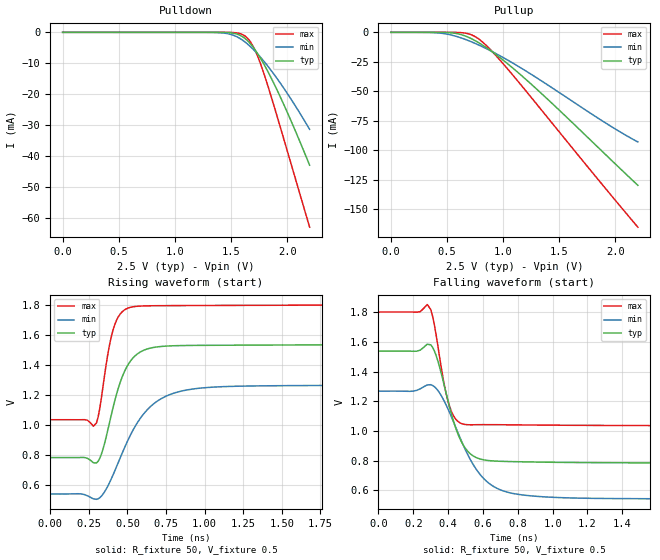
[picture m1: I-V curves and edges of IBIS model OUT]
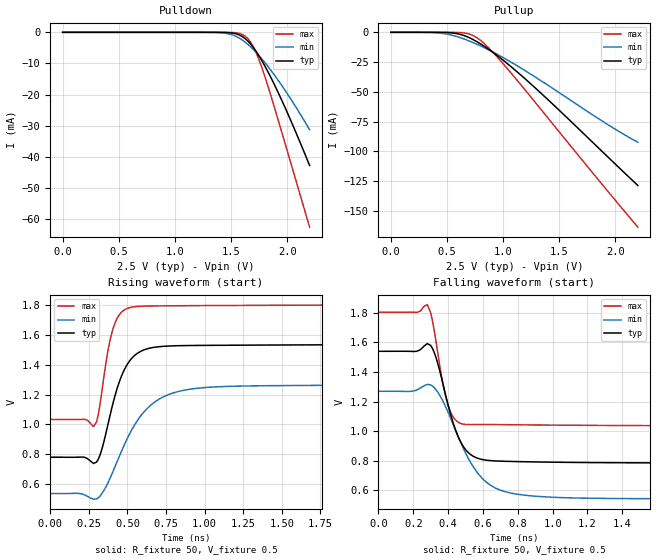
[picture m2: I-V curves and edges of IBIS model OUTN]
|   IBIS File of SG2520EHN D
|   LV-PECL, Vcc=2.5V, fo>212.5MHz
[IBIS Ver]   3.2
[File Name]   sg2520ehn_hf_25v.ibs
[File Rev]   1.0
[Date]   July 28, 2020
[Source]
[Notes]
Created by Minoru Kozaki
[Disclaimer]
Seiko Epson Corporation makes no warranty with respect to the
information contained herein.
[Copyright]
Copyright(C) 2020, Seiko Epson Corporation. All rights reserved.
|   Component
[Component]   SG2520EHN
[Manufacturer]  Seiko Epson Corporation
[Package]
R_pkg   17.7m   NA   NA
L_pkg   235p   NA   NA
C_pkg   208f   NA   NA
[Pin]   signal_name   model_name   R_pin   L_pin   C_pin
1   OE/ST   NC
2   NC   NC
3   GND   GND
4   OUT   OUT   17.7m   235p   208f
5   OUTN   OUTN   10.4m   129p   221f
6   VCC   POWER
[Diff Pin] inv_pin  vdiff  tdelay_typ
4   5   0   0
| Models and submodels in the file (2): OUT (Output_ECL), OUTN (Output_ECL)
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|   Model OUT
[Model]   OUT
Model_type   Output_ECL
Polarity   Non-Inverting
Vref = 0.5
Vmeas = 1.166
Rref = 50
Cref = 0
C_comp   0.5p   0.5p   0.5p
[Temperature Range]   25   105   -40
[Voltage Range]   2.5   2.25   2.75
[Pullup Reference]   2.5   2.25   2.75
[Pulldown Reference]   2.5   2.25   2.75
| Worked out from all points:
|   falling waveform, R_fixture 50, V_fixture 0.5: 20-80 % time 113ps typ, 191ps min, 71.9ps max; typ from 1.54 V to 0.783 V
|   rising waveform, R_fixture 50, V_fixture 0.5: 20-80 % time 131ps typ, 236ps min, 79.5ps max; typ from 0.782 V to 1.54 V
[Pullup]
0V        16.83nA    9.982nA    69.1nA
375mV     -8.971uA   -228.7uA   -2.724uA
550mV     -540.9uA   -2.566mA   -30.5uA
625mV     -1.913mA   -4.697mA   -262.1uA
700mV     -4.591mA   -7.353mA   -1.495mA
750mV     -7.012mA   -9.352mA   -3.594mA
800mV     -9.818mA   -11.5mA    -6.9mA
875mV     -14.57mA   -14.98mA   -13.49mA
950mV     -19.82mA   -18.72mA   -21.14mA
1.25V     -43.87mA   -35.56mA   -55.08mA
1.9V      -102.4mA   -75.99mA   -130.8mA
2.2V      -129.5mA   -92.83mA   -165mA
[Pulldown]
0V        16.83nA    9.981nA    69.1nA
1.4V      -16.08uA   -122.2uA   -3.959uA
1.55V     -538.1uA   -1.399mA   -182.6uA
1.625V    -1.987mA   -3.13mA    -1.2mA
1.675V    -3.792mA   -4.698mA   -3.188mA
1.7V      -4.94mA    -5.585mA   -4.749mA
1.725V    -6.23mA    -6.533mA   -6.681mA
1.775V    -9.163mA   -8.583mA   -11.44mA
1.85V     -14.21mA   -11.98mA   -19.88mA
1.95V     -21.76mA   -17.01mA   -32.04mA
2.075V    -32.05mA   -23.92mA   -47.53mA
2.2V      -42.98mA   -31.38mA   -63.01mA
[Falling Waveform]
R_fixture = 50
V_fixture = 0.5
V_fixture_min = 0.25
V_fixture_max = 0.75
0s        1.54V      1.27V      1.803V
280ps     1.586V     1.312V     1.854V
300ps     1.582V     1.313V     1.821V
330ps     1.513V     1.29V      1.655V
380ps     1.296V     1.197V     1.299V
410ps     1.154V     1.12V      1.16V
500ps     882.4mV    872mV      1.045V
650ps     800mV      635.1mV    1.044V
900ps     791.9mV    561.4mV    1.041V
4ns       782.5mV    540.4mV    1.035V
[Rising Waveform]
R_fixture = 50
V_fixture = 0.5
V_fixture_min = 0.25
V_fixture_max = 0.75
0s        781.5mV    539.1mV    1.034V
300ps     746mV      503.1mV    1.014V
340ps     832.7mV    535.5mV    1.244V
380ps     997.6mV    606.2mV    1.512V
410ps     1.129V     673.9mV    1.643V
470ps     1.33V      821mV      1.757V
530ps     1.439V     952.8mV    1.785V
710ps     1.521V     1.169V     1.794V
1ns       1.53V      1.247V     1.795V
4ns       1.538V     1.268V     1.802V
[Ramp]
R_load = 50
dV/dt_r   0.45153/130.10p   0.43527/234.73p   0.45877/78.94p
dV/dt_f   0.45153/112.26p   0.43527/189.43p   0.45877/71.26p
|   Model OUTN
[Model]   OUTN
Model_type   Output_ECL
Polarity   Inverting
Vref = 0.5
Vmeas = 1.166
Rref = 50
Cref = 0
C_comp   0.5p   0.5p   0.5p
[Temperature Range]   25   105   -40
[Voltage Range]   2.5   2.25   2.75
[Pullup Reference]   2.5   2.25   2.75
[Pulldown Reference]   2.5   2.25   2.75
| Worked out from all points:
|   falling waveform, R_fixture 50, V_fixture 0.5: 20-80 % time 113ps typ, 192ps min, 71.8ps max; typ from 1.54 V to 0.782 V
|   rising waveform, R_fixture 50, V_fixture 0.5: 20-80 % time 131ps typ, 237ps min, 79.4ps max; typ from 0.781 V to 1.54 V
[Pullup]
0V        16.83nA    9.981nA    69.09nA
375mV     -8.971uA   -228.6uA   -2.724uA
550mV     -540.6uA   -2.563mA   -30.5uA
625mV     -1.911mA   -4.689mA   -262uA
700mV     -4.581mA   -7.338mA   -1.493mA
750mV     -6.992mA   -9.331mA   -3.584mA
800mV     -9.787mA   -11.48mA   -6.871mA
875mV     -14.52mA   -14.94mA   -13.42mA
950mV     -19.74mA   -18.66mA   -21.02mA
1.25V     -43.66mA   -35.43mA   -54.7mA
1.9V      -101.8mA   -75.65mA   -129.9mA
2.2V      -128.8mA   -92.43mA   -163.8mA
[Pulldown]
0V        16.83nA    9.98nA     69.1nA
1.4V      -16.08uA   -122.2uA   -3.959uA
1.55V     -537.8uA   -1.398mA   -182.5uA
1.625V    -1.984mA   -3.125mA   -1.198mA
1.675V    -3.783mA   -4.689mA   -3.179mA
1.7V      -4.927mA   -5.575mA   -4.731mA
1.725V    -6.213mA   -6.519mA   -6.651mA
1.775V    -9.132mA   -8.564mA   -11.37mA
1.85V     -14.16mA   -11.95mA   -19.75mA
1.95V     -21.67mA   -16.96mA   -31.82mA
2.075V    -31.91mA   -23.84mA   -47.2mA
2.2V      -42.77mA   -31.28mA   -62.57mA
[Falling Waveform]
R_fixture = 50
V_fixture = 0.5
V_fixture_min = 0.25
V_fixture_max = 0.75
0s        1.539V     1.269V     1.802V
220ps     1.539V     1.278V     1.801V
280ps     1.591V     1.315V     1.854V
300ps     1.578V     1.312V     1.797V
330ps     1.497V     1.28V      1.606V
400ps     1.175V     1.126V     1.172V
490ps     891.6mV    877.3mV    1.047V
640ps     801.8mV    638.1mV    1.045V
900ps     792.5mV    561.5mV    1.042V
4ns       782.3mV    540.2mV    1.034V
[Rising Waveform]
R_fixture = 50
V_fixture = 0.5
V_fixture_min = 0.25
V_fixture_max = 0.75
0s        781.3mV    538.9mV    1.034V
280ps     739.7mV    500.2mV    985mV
300ps     749mV      503.1mV    1.018V
330ps     820.2mV    532.1mV    1.19V
370ps     983.5mV    603.3mV    1.47V
410ps     1.156V     695.4mV    1.651V
530ps     1.444V     968.3mV    1.784V
710ps     1.52V      1.172V     1.792V
1ns       1.528V     1.246V     1.794V
4ns       1.537V     1.267V     1.801V
[Ramp]
R_load = 50
dV/dt_r   0.45112/130.90p   0.43489/236.45p   0.45831/78.98p
dV/dt_f   0.45112/112.46p   0.43489/190.22p   0.45831/71.06p
